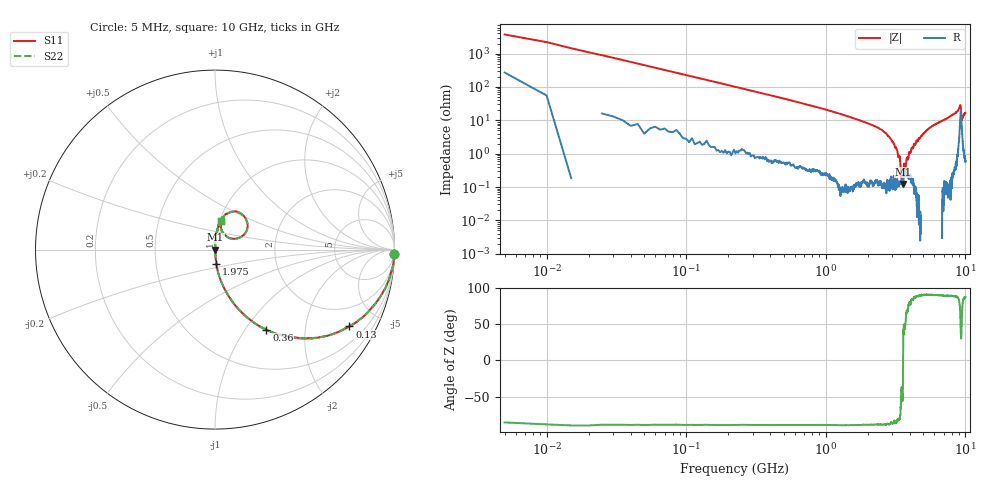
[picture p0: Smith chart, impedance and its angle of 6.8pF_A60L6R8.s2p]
! Amotech Co.,Ltd.
! http://www.amotech.co.kr/
! Part Number: A60L6R8
! These Parameters are Measured in Series Mode Connection
! Operation Temp=25[degC], DC Bias Voltage=0[V]
! Freq. Start=5[MHz] Stop=10[GHz], 2000[Steps]
! Date: Monday, July 14, 2020, 09:33:31
# GHZ S RI R 50.000000
!Freq.(Hz) S11(Real) S11(Imag) S21(Real) S21(Imag) S12(Real) S12(Imag) S22(Real) S22(Imag)
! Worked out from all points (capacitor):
!   2000 points, 5 MHz to 10 GHz, reference 50 ohm
!   read as one part in series: C = 7.05 pF near 55 MHz
!   lowest |Z| = 123 mohm at 3.57 GHz (marker M1)
!   series resonance near 3.579 GHz, so ESL is about 280 pH
!   S11 on the Smith chart (normalised r, x): 5 MHz: 6, -75; 130 MHz: 1.04, -3.48; 360 MHz: 1.01, -1.26; 1.975 GHz: 1.00, -0.17; 10 GHz: 1.01, +0.33
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0.005  0.9974 -0.0265  0.00264 0.0265  0.00264 0.0265  0.9974 -0.0265
0.07  0.9079 -0.2804  0.0921 0.2804  0.0921 0.2804  0.9079 -0.2804
0.13  0.7491 -0.4283  0.2509 0.4283  0.2509 0.4283  0.7491 -0.4283
0.36  0.2866 -0.4464  0.7134 0.4464  0.7134 0.4464  0.2866 -0.4464
0.755  0.0796 -0.2653  0.9204 0.2653  0.9204 0.2653  0.0796 -0.2653
1.675  0.0124 -0.1046  0.9876 0.1046  0.9876 0.1046  0.0124 -0.1046
1.975  0.00797 -0.0819  0.992 0.0819  0.992 0.0819  0.00797 -0.0819
2.865  0.00201 -0.031  0.998 0.031  0.998 0.031  0.00201 -0.031
3.34  0.00135 -0.0076  0.9987 0.0076  0.9987 0.0076  0.00135 -0.0076
3.395  0.00152 -0.0069  0.9985 0.0069  0.9985 0.0069  0.00152 -0.0069
3.48  0.00144 -0.00127  0.9986 0.00127  0.9986 0.00127  0.00144 -0.00127
3.57  0.00109 -0.000572  0.9989 0.000572  0.9989 0.000572  0.00109 -0.000572
3.645  0.00336 0.00334  0.9966 -0.00334  0.9966 -0.00334  0.00336 0.00334
3.72  0.00234 0.00279  0.9977 -0.00279  0.9977 -0.00279  0.00234 0.00279
3.81  0.00277 0.00698  0.9972 -0.00698  0.9972 -0.00698  0.00277 0.00698
3.98  0.0023 0.0105  0.9977 -0.0105  0.9977 -0.0105  0.0023 0.0105
5.005  0.00102 0.0398  0.999 -0.0398  0.999 -0.0398  0.00102 0.0398
6.67  0.00826 0.0919  0.9917 -0.0919  0.9917 -0.0919  0.00826 0.0919
8.335  0.0269 0.1523  0.9731 -0.1523  0.9731 -0.1523  0.0269 0.1523
9.185  0.1516 0.1958  0.8484 -0.1958  0.8484 -0.1958  0.1516 0.1958
9.43  0.0579 0.079  0.9421 -0.079  0.9421 -0.079  0.0579 0.079
10  0.0324 0.1607  0.9676 -0.1607  0.9676 -0.1607  0.0324 0.1607
